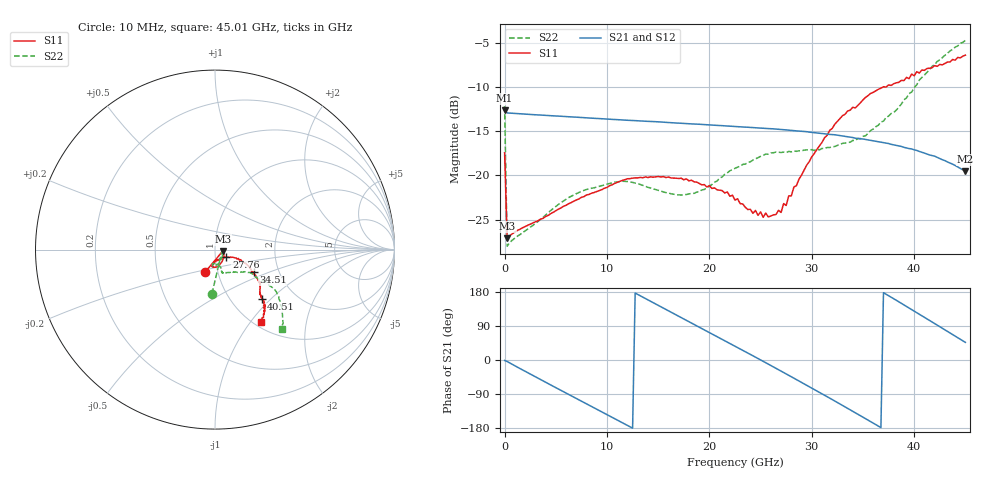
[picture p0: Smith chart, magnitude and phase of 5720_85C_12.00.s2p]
! Device:  ADRF5720
! Description: 0.5dB LSB GaAs MMIC 6-bit Digital Attenuator
! Frequency:  0.000009 -  40 GHz
! Ports:
!	RF1	= Port 1
!	RF2	= Port 2
! Vdd:  3.3 Volt
! Vss:  -3.3 Volt
! Control:  0/3.3 Volt
! State:  12.00 dB attenuation
! Data:  The device was measured using G-S-G Probes on a matrix board.
!  Data was collected using an calibrated 4 port network analyzer.
!  The reference plane for this measurement is at the launchers.
! Note:  Analog Devices supplies this data as a sample of measured data
!  for this product.  Your particular data for this product may vary.
!  Data was taken at 85 degrees C.
!  Analog Devices reserves the right to change this data at anytime.
# GHZ S DB R 45.0
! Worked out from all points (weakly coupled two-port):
!   181 points, 10 MHz to 45.01 GHz, reference 45 ohm
!   highest |S21| = -12.62 dB at 10 MHz (marker M1); lowest = -19.5 dB at 45.01 GHz (marker M2)
!   lowest |S11| = -27.1 dB at 260 MHz (marker M3), VSWR 1.09, Z = 49.1 - j0.842 ohm
!   |S11| at or under -10 dB: start of sweep to 36.96 GHz; 37.1975 GHz to 37.27042 GHz (72.92 MHz wide, 0.196 % of centre)
!   |S22| runs from -28.0 to -4.7 dB; largest |S21 - S12| = 0.001
!   S11 on the Smith chart (normalised r, x): 10 MHz: 0.87, -0.22; 27.76 GHz: 1.13, -0.10; 34.51 GHz: 1.48, -0.40; 40.51 GHz: 1.37, -0.89; 45.01 GHz: 1.07, -1.12
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0.01  -17.44 -113.5  -12.62 -1.2  -12.61 -1.2  -12.15 -94.0
0.26  -27.12 -11.2  -12.93 -4.0  -12.92 -4.0  -27.99 -12.7
4.26  -24.52 -35.4  -13.22 -62.2  -13.21 -62.2  -24.23 -52.7
7.76  -22.39 -58.2  -13.46 -112.3  -13.45 -112.2  -21.69 -78.5
11.51  -20.55 -78.7  -13.72 -165.6  -13.71 -165.5  -20.65 -96.0
15.26  -20.17 -93.5  -13.96 140.8  -13.94 141.0  -21.77 -99.5
19.01  -20.89 -99.6  -14.21 87.1  -14.19 87.3  -21.82 -81.7
22.76  -22.63 -92.8  -14.48 32.9  -14.47 33.1  -19.06 -72.0
25.26  -24.73 -74.4  -14.66 -3.5  -14.65 -3.2  -17.72 -72.7
27.01  -24.18 -45.5  -14.80 -29.3  -14.78 -29.1  -17.40 -71.8
27.26  -23.17 -40.4  -14.83 -33.1  -14.81 -32.9  -17.36 -72.2
27.51  -23.39 -38.4  -14.85 -36.8  -14.84 -36.5  -17.41 -71.4
27.76  -22.30 -34.2  -14.88 -40.5  -14.86 -40.2  -17.28 -72.1
28.01  -22.31 -33.8  -14.90 -44.3  -14.89 -44.0  -17.33 -71.5
30.26  -17.50 -23.1  -15.16 -77.9  -15.14 -77.7  -17.18 -68.0
33.01  -13.24 -27.0  -15.54 -120.0  -15.53 -119.8  -16.37 -57.5
34.51  -12.08 -30.4  -15.82 -142.9  -15.80 -142.6  -15.81 -51.4
35.76  -10.72 -34.9  -16.02 -162.7  -16.00 -162.4  -14.92 -45.1
37.76  -9.82 -39.3  -16.48 165.5  -16.46 165.8  -13.00 -34.7
40.51  -8.42 -46.8  -17.28 120.6  -17.27 121.0  -9.22 -32.6
42.26  -7.67 -49.2  -17.95 92.0  -17.92 92.3  -7.11 -36.4
45.01  -6.40 -58.0  -19.52 46.6  -19.49 46.9  -4.74 -50.0
